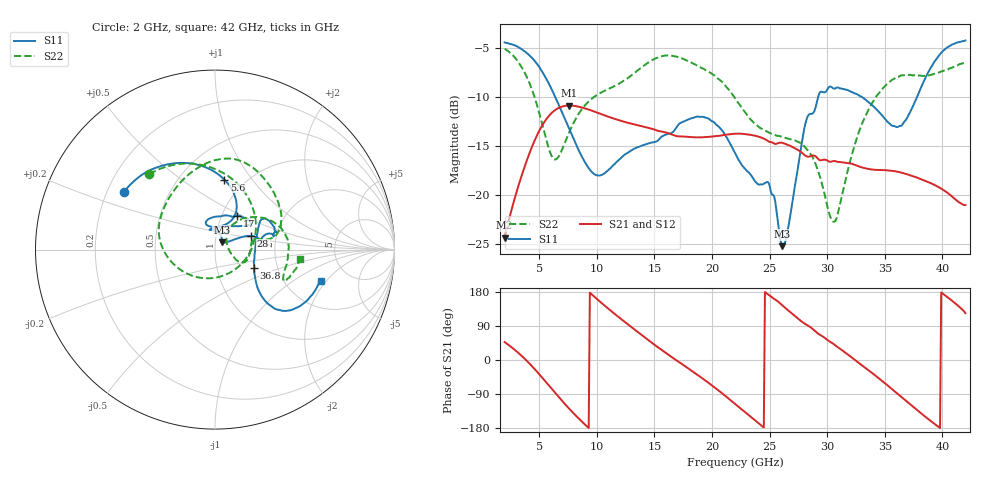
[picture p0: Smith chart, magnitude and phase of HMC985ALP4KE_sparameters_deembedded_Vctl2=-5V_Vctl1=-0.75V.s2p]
!s2p File: Measurements: S11, S21, S12, S22
# GHz S dB R 50.0
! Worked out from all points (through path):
!   401 points, 2 GHz to 42 GHz, reference 50 ohm
!   highest |S21| = -10.87 dB at 7.6 GHz (marker M1); lowest = -24.4 dB at 2 GHz (marker M2)
!   lowest |S11| = -25.2 dB at 26.1 GHz (marker M3), VSWR 1.12, Z = 53.7 + j4.3 ohm
!   |S11| at or under -10 dB: 6.397 GHz to 29.22 GHz (22.82 GHz wide, 128 % of centre); 33.03 GHz to 37.8 GHz (4.772 GHz wide, 13.5 % of centre)
!   |S22| runs from -22.7 to -5.1 dB; largest |S21 - S12| = 0.00031
!   S11 on the Smith chart (normalised r, x): 2 GHz: 0.27, +0.27; 5.6 GHz: 0.80, +0.74; 17 GHz: 1.18, +0.47; 28 GHz: 1.48, +0.24; 36.8 GHz: 1.51, -0.33; 42 GHz: 3.11, -1.76
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2  -4.43 147.4  -24.36 47.4  -24.37 47.4  -5.07 131.0
3.6  -5.22 120.8  -17.59 7.4  -17.59 7.4  -7.21 86.0
4.7  -6.45 100.0  -14.19 -27.0  -14.19 -27.0  -10.38 44.3
5.6  -8.10 82.4  -12.29 -58.6  -12.30 -58.6  -14.28 -5.5
6.4  -10.01 69.3  -11.31 -87.3  -11.32 -87.3  -16.38 -68.4
7.6  -13.24 59.8  -10.87 -128.4  -10.87 -128.4  -13.62 -141.4
8.7  -16.07 65.6  -11.06 -162.3  -11.06 -162.3  -11.24 -174.0
11.9  -16.43 109.3  -12.36 113.2  -12.36 113.3  -8.66 139.6
15.4  -14.33 77.8  -13.47 31.7  -13.48 31.7  -5.92 86.3
17  -12.96 57.0  -14.00 -2.7  -14.01 -2.7  -5.91 67.4
19.6  -12.15 35.4  -14.07 -58.0  -14.08 -58.0  -7.36 32.3
22  -15.70 52.8  -13.74 -115.7  -13.75 -115.6  -10.11 11.1
24.9  -18.71 99.4  -14.52 172.3  -14.53 172.3  -13.60 12.0
26.1  -25.21 46.6  -14.68 144.5  -14.68 144.5  -14.06 -1.1
28  -13.30 20.7  -15.88 96.9  -15.88 96.9  -15.01 -23.5
28.7  -11.70 11.0  -15.97 82.9  -15.98 82.9  -16.06 -26.7
30.7  -9.12 18.8  -16.54 38.7  -16.54 38.7  -22.66 24.9
32.9  -9.92 32.4  -17.14 -11.3  -17.15 -11.3  -13.10 49.3
35.4  -12.68 10.1  -17.50 -71.0  -17.50 -71.0  -8.48 20.8
36.8  -12.38 -25.0  -17.84 -106.7  -17.84 -106.6  -7.74 3.7
39.6  -5.94 -42.4  -19.14 -175.0  -19.14 -174.9  -7.54 -24.3
42  -4.23 -16.6  -21.02 123.3  -21.02 123.4  -6.43 -6.2
